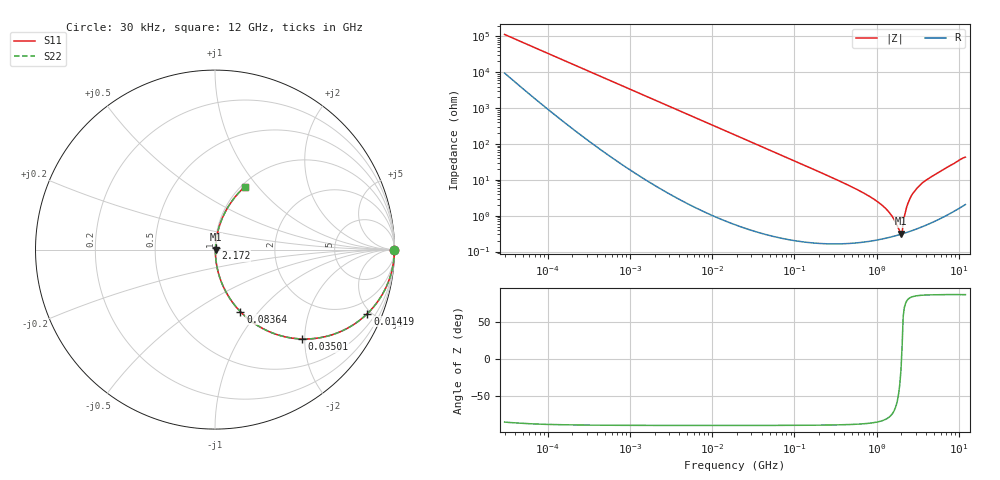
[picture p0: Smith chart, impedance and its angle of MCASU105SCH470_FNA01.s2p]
! MCASU105SCH470_FNA01  S-PARAMETER MODEL  ( General Type )
! Model Generated by TAIYO YUDEN Corporation (http://www.ty-top.com)
! Version 1.0
! TAIYO YUDEN Control No. 130207
! Copyright(c) 2013 TAIYO YUDEN CO.,LTD. All Rights Reserved.
! Product Description (link to TY-COMPAS)
! https://ds.yuden.co.jp/TYCOMPAS/or/detail?pn=MCASU105SCH470JFNA01&u=M
! Products Name : Multilayer Ceramic Capacitors
! Characteristics :
!  Capacitance : 47 pF , Rated Voltage : 50V , TCC : CH / C0H
!  Case Size : 1.0 x 0.5 / 0.039 x 0.02 [mm/inch] , Thickness : 0.5 / 0.02 [mm/inch]
!  (Conditions: Temperature = 25 degC , DC Bias Current/Voltage = 0A / 0V)
! External Node Assignments :
!  1  o---| |---o  2
! GND o---------o GND
! Frequency Range : 30000Hz  -  12GHz  [ 401 STEP ]
# MHz S RI R 50
! Freq[MHz].  S11 Real  S11 Imag  S21 Real  S21 Imag  S12 Real  S12 Imag  S22 Real  S22 Imag
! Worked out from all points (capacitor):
!   401 points, 30 kHz to 12 GHz, reference 50 ohm
!   read as one part in series: C = 47.1 pF near 32 kHz
!   lowest |Z| = 317 mohm at 1.972 GHz (marker M1)
!   series resonance near 2.006 GHz, so ESL is about 130 pH
!   S11 on the Smith chart (normalised r, x): 30 kHz: open; 14.19 MHz: 1.01, -4.76; 35.01 MHz: 1.01, -1.93; 83.64 MHz: 1.00, -0.81; 2.172 GHz: 1.01, +0.02; 12 GHz: 1.04, +0.86
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0.03  0.9999 -0.000881  7.48e-05 0.000881  7.48e-05 0.000881  0.9999 -0.000881
0.260295  0.9998 -0.0077  0.000159 0.0077  0.000159 0.0077  0.9998 -0.0077
2.258455  0.9953 -0.0665  0.00471 0.0665  0.00471 0.0665  0.9953 -0.0665
6.982189  0.9585 -0.1979  0.0415 0.1979  0.0415 0.1979  0.9585 -0.1979
14.194  0.8492 -0.3563  0.1508 0.3563  0.1508 0.3563  0.8492 -0.3563
18.97367  0.7596 -0.4258  0.2404 0.4258  0.2404 0.4258  0.7596 -0.4258
35.01459  0.4821 -0.4979  0.5179 0.4979  0.5179 0.4979  0.4821 -0.4979
83.63502  0.1413 -0.3456  0.8587 0.3456  0.8587 0.3456  0.1413 -0.3456
164.6252  0.0415 -0.1951  0.9585 0.1951  0.9585 0.1951  0.0415 -0.1951
725.66  0.00349 -0.0404  0.9965 0.0404  0.9965 0.0404  0.00349 -0.0404
1068.55  0.00266 -0.0228  0.9973 0.0228  0.9973 0.0228  0.00266 -0.0228
1428.372  0.00262 -0.0119  0.9974 0.0119  0.9974 0.0119  0.00262 -0.0119
1625.032  0.00273 -0.00746  0.9973 0.00746  0.9973 0.00746  0.00273 -0.00746
1909.359  0.00297 -0.00206  0.997 0.00206  0.997 0.00206  0.00297 -0.00206
1971.936  0.00303 -0.000889  0.997 0.000889  0.997 0.000889  0.00303 -0.000889
2036.564  0.0031 0.0008  0.9969 -0.0008  0.9969 -0.0008  0.0031 0.0008
2172.242  0.00332 0.00882  0.9967 -0.00882  0.9967 -0.00882  0.00332 0.00882
2316.96  0.00369 0.0169  0.9963 -0.0169  0.9963 -0.0169  0.00369 0.0169
2552.314  0.00457 0.0301  0.9954 -0.0301  0.9954 -0.0301  0.00457 0.0301
3303.507  0.00906 0.0669  0.9909 -0.0669  0.9909 -0.0669  0.00906 0.0669
4710.119  0.0215 0.1215  0.9785 -0.1215  0.9785 -0.1215  0.0215 0.1215
12000  0.1669 0.3497  0.8331 -0.3497  0.8331 -0.3497  0.1669 0.3497
